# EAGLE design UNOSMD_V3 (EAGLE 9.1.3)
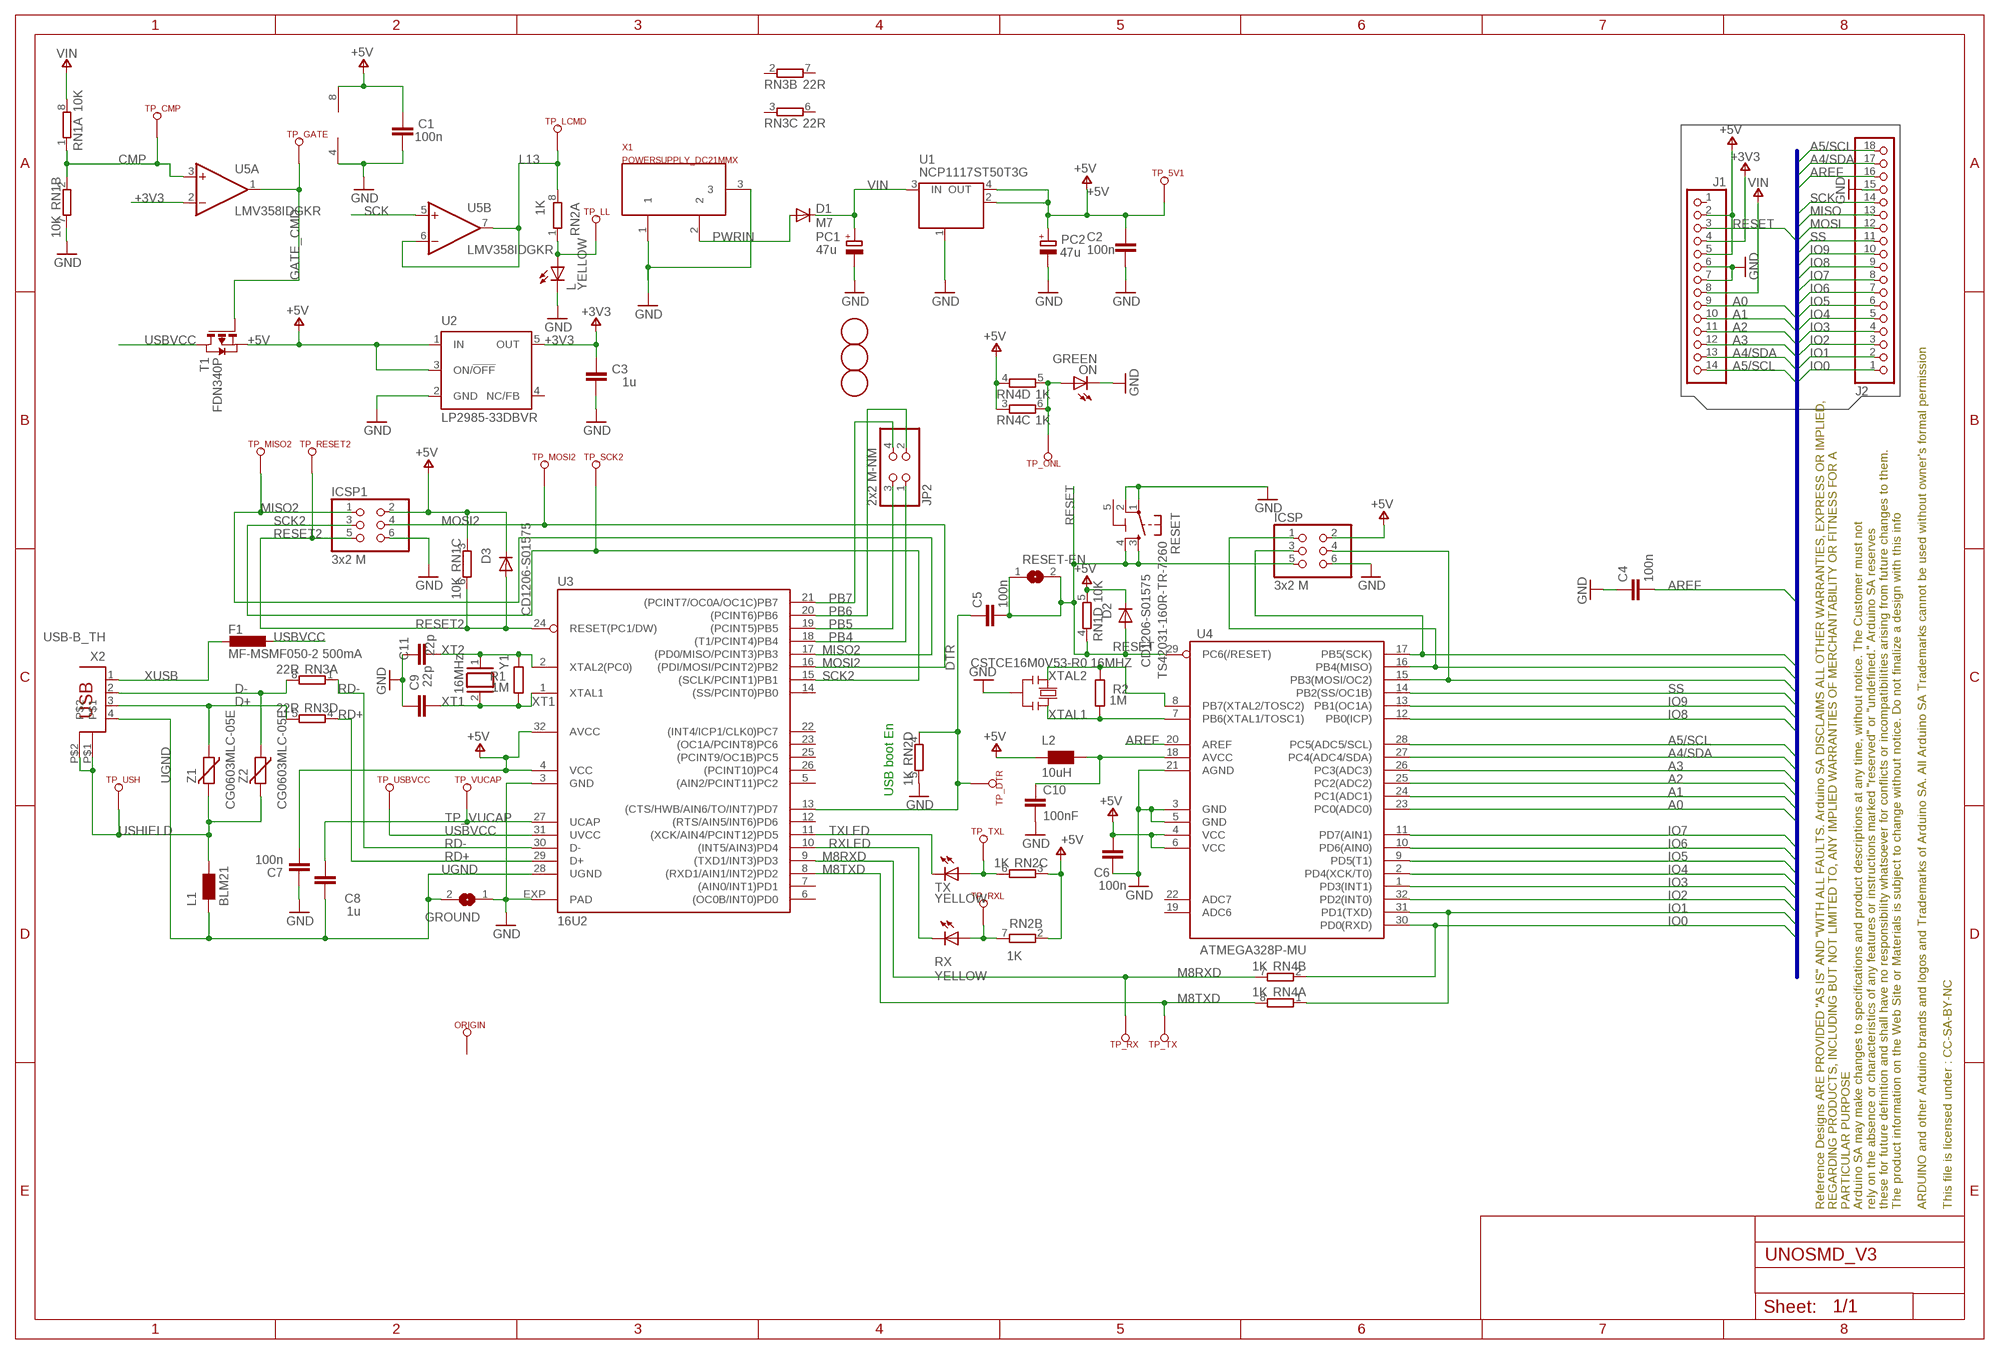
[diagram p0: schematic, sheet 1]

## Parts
C1  100n  C-EU0603-RND  [C0603-ROUND]
C2  100n  C-EU0603-RND  [C0603-ROUND]
C3  1u  C-EU0603-RND  [C0603-ROUND]
C4  100n  C-EU0603-RND  [C0603-ROUND]
C5  100n  C-EU0603-RND  [C0603-ROUND]
C6  100n  C-EU0603-RND  [C0603-ROUND]
C7  100n  C-EU0603-RND  [C0603-ROUND]
C8  1u  C-EU0603-RND  [C0603-ROUND]
C9  22p  C-EU0603-RND  [C0603-ROUND]
C10  100nF  0015_100NF_0603  [C0603-ROUND]
C11  22p  C-EU0603-RND  [C0603-ROUND]
D1  M7  DIODE-SMB  [SMB]
D2  CD1206-S01575  DIODE-MINIMELF  [MINIMELF]
D3  CD1206-S01575  DIODE-MINIMELF  [MINIMELF]
F1  MF-MSMF050-2 500mA  L-EUL1812  [L1812]
FD1  DNP  FIDUCIAL-1.5MM  [FD-1-1.5]
FD2  DNP  FIDUCIAL-1.5MM  [FD-1-1.5]
FD3  DNP  FIDUCIAL-1.5MM  [FD-1-1.5]
FRAME1  DNP  A3-FRAME-STANDARD  [FRAME]
GROUND  SJ  [SJ]
ICSP  3x2 M  PINHD-2X3  [2X03]
ICSP1  3x2 M  PINHD-2X3  [2X03]
J1  -  PINHD-1X14-CUSTOM  [1X14-CUSTOM]
J2  -  PINHD-1X18  [1X18-CUSTOM]
JP2  2x2 M-NM  PINHD-2X2  [2X02]
L  YELLOW  LEDCHIP-LED0805  [CHIP-LED0805]
L1  BLM21  WE-CBF_0805  [0805]
L2  10uH  0715_CV201210-100K  [0805]
ON  GREEN  LEDCHIP-LED0805  [CHIP-LED0805]
ORIGIN  TP_SP  [TP-SP]
PC1  47u  CPOL-EUD  [PANASONIC_D]
PC2  47u  CPOL-EUD  [PANASONIC_D]
R1  1M  R-EU_R0603  [R0603-ROUND]
R2  1M  R-EU_R0603  [R0603-ROUND]
RESET  TS42031-160R-TR-7260  TS42  [TS42]
RESET-EN  SJ  [SJ]
RN1  10K  4R-NCAY16  [CAY16]
RN2  1K  4R-NCAY16  [CAY16]
RN3  22R  4R-NCAY16  [CAY16]
RN4  1K  4R-NCAY16  [CAY16]
RX  YELLOW  LEDCHIP-LED0805  [CHIP-LED0805]
T1  FDN340P  PMOSSOT23  [SOT-23]
TP_5V1  TP_SP  [TP-SP]
TP_CMP  TP_SP  [TP-SP]
TP_DTR  TP_SP  [TP-SP]
TP_GATE  TP_SP  [TP-SP]
TP_LCMD  TP_SP  [TP-SP]
TP_LL  TP_SP  [TP-SP]
TP_MISO2  TP_SP  [TP-SP]
TP_MOSI2  TP_SP  [TP-SP]
TP_ONL  TP_SP  [TP-SP]
TP_RESET2  TP_SP  [TP-SP]
TP_RX  TP_SP  [TP-SP]
TP_RXL  TP_SP  [TP-SP]
TP_SCK2  TP_SP  [TP-SP]
TP_TX  TP_SP  [TP-SP]
TP_TXL  TP_SP  [TP-SP]
TP_USBVCC  TP_SP  [TP-SP]
TP_USH  TP_SP  [TP-SP]
TP_VUCAP  TP_SP  [TP-SP]
TX  YELLOW  LEDCHIP-LED0805  [CHIP-LED0805]
U1  NCP1117ST50T3G  MC33269ST-3.3T3  [SOT223]
U2  LP2985-33DBVR  LP2985-XXDBVR33  [SOT23-DBV]
U3  16U2  ATMEGA16U2  [ATMEL_QFN32]
U4  ATMEGA328P-MU  ATMEGAXX8-MUR  [MLF32]
U5  LMV358IDGKR  LMV358MMX  [MSOP08]
X1  POWERSUPPLY_DC21MMX  [POWERSUPPLY_DC-21MM]
X2  USB-B_TH  PN61729  [PN61729]
Y1  16MHz  XTAL/S  [QS]
Y2  CSTCE16M0V53-R0 16MHZ  RESONATORMU  [RESONATOR]
Z1  CG0603MLC-05E  VARISTORCN0603  [CT/CN0603]
Z2  CG0603MLC-05E  VARISTORCN0603  [CT/CN0603]

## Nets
+3V3: C3.2 J1.4 U2.5(OUT) U5.2(A:-IN)
+5V [usbvcc]: C1.2 C2.2 C6.2 C7.1 D2.C D3.C ICSP1.2 ICSP.2 J1.2 J1.5 L2.1 PC2.+ RN1.3 RN1.5 RN2.2 RN2.3 RN4.3 RN4.4 T1.2(S) TP_5V1.X(TESTP) U1.2(OUT) U1.4(OUT) U2.1(IN) U2.3(ON/!OFF) U3.4(VCC) U3.32(AVCC) U4.4(VCC) U4.6(VCC) U5.8(P:V+)
A0: J1.9 U4.23(PC0(ADC0))
A1: J1.10 U4.24(PC1(ADC1))
A2: J1.11 U4.25(PC2(ADC2))
A3: J1.12 U4.26(PC3(ADC3))
A4/SDA: J1.13 J2.17 U4.27(PC4(ADC4/SDA))
A5/SCL: J1.14 J2.18 U4.28(PC5(ADC5/SCL))
AREF [aref]: C4.2 J2.16 U4.20(AREF)
CMP: RN1.1 RN1.2 TP_CMP.X(TESTP) U5.3(A:+IN)
D+: RN3.5 X2.3 Z1.1
D-: RN3.8 X2.2 Z2.1
DTR: C5.1 RN2.4 TP_DTR.X(TESTP) U3.13((CTS/HWB/AIN6/TO/INT7)PD7)
GATE_CMD: T1.3(G) TP_GATE.X(TESTP) U5.1(A:OUT)
GND [gnd]: C1.1 C2.1 C3.1 C4.1 C6.1 C7.2 C9.2 C10.2 C11.2 GROUND.1 ICSP1.6 ICSP.6 J1.6 J1.7 J2.15 L.C ON.C PC1.- PC2.- RESET.1 RESET.2 RN1.7 RN2.5 U1.1(GND/ADJ) U2.2(GND) U3.3(GND) U3.EXP(PAD) U4.3(GND) U4.5(GND) U4.21(AGND) U5.4(P:V-) X1.1 X1.3 Y2.2
IO0: J2.1 RN4.2 U4.30(PD0(RXD))
IO1: J2.2 RN4.1 U4.31(PD1(TXD))
IO2: J2.3 U4.32(PD2(INT0))
IO3: J2.4 U4.1(PD3(INT1))
IO4: J2.5 U4.2(PD4(XCK/T0))
IO5: J2.6 U4.9(PD5(T1))
IO6: J2.7 U4.10(PD6(AIN0))
IO7: J2.8 U4.11(PD7(AIN1))
IO8: J2.9 U4.12(PB0(ICP))
IO9: J2.10 U4.13(PB1(OC1A))
L13: RN2.8 TP_LCMD.X(TESTP) U5.6(B:-IN) U5.7(B:OUT)
M8RXD: RN4.7 TP_RX.X(TESTP) U3.9((TXD1/INT3)PD3)
M8TXD: RN4.8 TP_TX.X(TESTP) U3.8((RXD1/AIN1/INT2)PD2)
MISO: ICSP.1 J2.13 U4.16(PB4(MISO))
MISO2: ICSP1.1 TP_MISO2.X(TESTP) U3.17((PD0/MISO/PCINT3)PB3)
MOSI: ICSP.4 J2.12 U4.15(PB3(MOSI/OC2))
MOSI2: ICSP1.4 TP_MOSI2.X(TESTP) U3.16((PDI/MOSI/PCINT2)PB2)
N$1: L.A RN2.1 TP_LL.X(TESTP)
N$3: ON.A RN4.5 RN4.6 TP_ONL.X(TESTP)
N$4 [usbvcc]: C10.1 L2.2 U4.18(AVCC)
N$35: RN2.7 RX.A TP_RXL.X(TESTP)
N$36: RN2.6 TP_TXL.X(TESTP) TX.A
PB4: JP2.1 U3.18((T1/PCINT4)PB4)
PB5: JP2.3 U3.19((PCINT5)PB5)
PB6: JP2.2 U3.20((PCINT6)PB6)
PB7: JP2.4 U3.21((PCINT7/OC0A/OC1C)PB7)
PWRIN [power]: D1.A X1.2
RD+: RN3.4 U3.29(D+)
RD-: RN3.1 U3.30(D-)
RESET: C5.2 D2.A ICSP.5 J1.3 RESET-EN.1 RESET-EN.2 RESET.3 RESET.4 RN1.4 U4.29(PC6(/RESET))
RESET2: D3.A ICSP1.5 RN1.6 TP_RESET2.X(TESTP) U3.24(RESET(PC1/DW))
RXLED: RX.C U3.10((INT5/AIN3)PD4)
SCK: ICSP.3 J2.14 U4.17(PB5(SCK)) U5.5(B:+IN)
SCK2: ICSP1.3 TP_SCK2.X(TESTP) U3.15((SCLK/PCINT1)PB1)
SS: J2.11 U4.14(PB2(SS/OC1B))
TP_VUCAP: C8.1 TP_VUCAP.X(TESTP) U3.27(UCAP)
TXLED: TX.C U3.11((XCK/AIN4/PCINT12)PD5)
UGND [gnd]: C8.2 GROUND.2 L1.1 U3.28(UGND) X2.4
USBVCC [usbvcc]: F1.1 T1.1(D) TP_USBVCC.X(TESTP) U3.31(UVCC)
USHIELD [gnd]: L1.2 TP_USH.X(TESTP) X2.P$1 X2.P$2 Z1.2 Z2.2
VIN [power]: D1.C J1.8 PC1.+ RN1.8 U1.3(IN)
XT1: C9.1 R1.1 U3.1(XTAL1) Y1.2
XT2: C11.1 R1.2 U3.2(XTAL2(PC0)) Y1.1
XTAL1: R2.1 U4.7(PB6(XTAL1/TOSC1)) Y2.3
XTAL2: R2.2 U4.8(PB7(XTAL2/TOSC2)) Y2.1
XUSB [usbvcc]: F1.2 X2.1
Unconnected: J1.1 ORIGIN.X(TESTP) RN3.2 RN3.3 RN3.6 RN3.7 U2.4(NC/FB) U3.5((AIN2/PCINT11)PC2) U3.6((OC0B/INT0)PD0) U3.7((AIN0/INT1)PD1) U3.12((RTS/AIN5/INT6)PD6) U3.14((SS/PCINT0)PB0) U3.22((INT4/ICP1/CLK0)PC7) U3.23((OC1A/PCINT8)PC6) U3.25((PCINT9/OC1B)PC5) U3.26((PCINT10)PC4) U4.19(ADC6) U4.22(ADC7)

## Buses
B$1

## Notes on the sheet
- USB boot En

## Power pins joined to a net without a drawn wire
5-GND: RESET.5(5-GND)

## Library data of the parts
C1-C9 C11 = SmartPrj:C-EU: CAPACITOR, European symbol
C10 = Condensatori:0015_100NF_0603: 100nF 0603; CASE: 0603; MONTHLY_USAGE: _____; PART_NUMBER: 100nF_0603; PRICE: _____; SUPPLIER: _____; TYPE: Condensatori
D1-D3 = diode:DIODE-: DIODE
F1 = rcl:L-EU: INDUCTOR, European symbol
FD1-FD3 = Arduino-utility:FIDUCIAL: Fiducial mount; DATASHEET: DNP; DISTRIBUTOR-LINK: DNP; DISTRIBUTOR-PN: DNP; MANUFACTURER: DNP; MANUFACTURER-PN: DNP
FRAME1 = Arduino-utility:A3-FRAME: Schematic frame; CODE-ARDUINO: DNP; DATASHEET: DNP; DISTRIBUTOR-LINK: DNP; DISTRIBUTOR-PN: DNP; MANUFACTURER: DNP; MANUFACTURER-PN: DNP
GROUND RESET-EN = jumper:SJ: SMD solder JUMPER
ICSP ICSP1 = SmartPrj:PINHD-2X3: PIN HEADER
J1 = Arduino-connectors:PINHD-1X14: PIN HEADER; DATASHEET: -; DISTRIBUTOR-PN: -; MANUFACTURER: -; MANUFACTURER-PN: -
J2 = Arduino-connectors:PINHD-1X18; DATASHEET: -; DISTRIBUTOR-LINK: -; DISTRIBUTOR-PN: -; MANUFACTURER-PN: -; MANUFCATURER: -
JP2 = SmartPrj:PINHD-2X2: PIN HEADER
L ON RX TX = led:LED: LED
L1 = wuerth-elektronik:WE-CBF: SMD EMI Suppression Ferrite Beads
L2 = Induttanze:0715_CV201210-100K: 10uH 0805; CASE: 0805; MONTHLY_USAGE: _____; PART_NUMBER: CV201210-100K; PRICE: _____; SUPPLIER: _____; TYPE: Induttanze
ORIGIN TP_5V1 TP_CMP TP_DTR TP_GATE TP_LCMD TP_LL TP_MISO2 TP_MOSI2 TP_ONL TP_RESET2 TP_RX TP_RXL TP_SCK2 TP_TX TP_TXL TP_USBVCC TP_USH TP_VUCAP = SmartPrj:TP_SP
PC1 PC2 = rcl:CPOL-EU: POLARIZED CAPACITOR, European symbol
R1 R2 = SmartPrj:R-EU_: RESISTOR, European symbol
RESET = SmartPrj:TS42: TS42 Dongnan Electronics Tact switch VDC 12V - 50mA
RN1-RN4 = resistor-dil:4R-N: Array Chip Resistor Source: RS Component / Phycomp
T1 = zetex:PMOSSOT23: MOS FET
U1 = linear:MC33269ST*: Adjustable Output Low Dropout Voltage Regulator 800 mA Source: http://www.onsemi.com/pub/Collateral/MC33269-D.PDF
U2 = SmartPrj:LP2985-XXDBVR: ULTRALOW-POWER 50-mA LOW-DROPOUT LINEAR REGULATORS 50-mA Low-Dropout Regulator Source: http://focus.ti.com/lit/ds/symlink/tps77001.pdf
U3 = Arduino-ucs&SoCs:ATMEGA16U2: AVR AVR® ATmega Microcontroller IC 8-Bit 16MHz 16KB (8K x 16) FLASH 32-VQFN (5x5); DATASHEET: http://www.digikey.com/product-detail/en/atmel/ATMEGA16U2-MU/ATMEGA16U2-MU-ND/2050821; DISTRIBUTOR-LINK: http://www.digikey.com/product-detail/en/atmel/ATMEGA16U2-MU/ATMEGA16U2-MU-ND/2050821; DISTRIBUTOR-PN: ATMEGA16U2-MU-ND; MANUFACTURER: ATMEL; MANUFACTURER-PN: ATMEGA16U2-MU
U4 = SmartPrj:ATMEGAXX8: MICROCONTROLLER 8 Kbytes FLASH 1 kbytes SRAM 512 bytes EEPROM USART 6-channel 10 bit ADC 2-channel 8 bit ADC Source: avr.lbr
U5 = linear:LMV358?*: Dual General Purpose, Low Voltage, Rail-to-Rail Output Operational Amplifiers Source: http://www.national.com/mpf/LM/LMV321.html http://www.national.com/dt/lmv_qual.pdf
X1 = SmartPrj:POWERSUPPLY_DC21MM
X2 = SmartPrj:PN61729: BERG USB connector
Y1 = SmartPrj:XTAL/S: CRYSTAL
Y2 = SmartPrj:RESONATOR
Z1 Z2 = varistor:VARISTOR: VARISTOR

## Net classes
0 default: width 0.254 mm, clearance 0.254 mm
1 power: width 0.61 mm, drill 0.61 mm, clearance 0.254 mm
2 gnd: width 0.305 mm, drill 0.559 mm, clearance 0.254 mm
3 usbvcc: width 0.508 mm, drill 0.61 mm, clearance 0.254 mm
4 aref: width 0.406 mm, drill 0.61 mm, clearance 0.254 mm

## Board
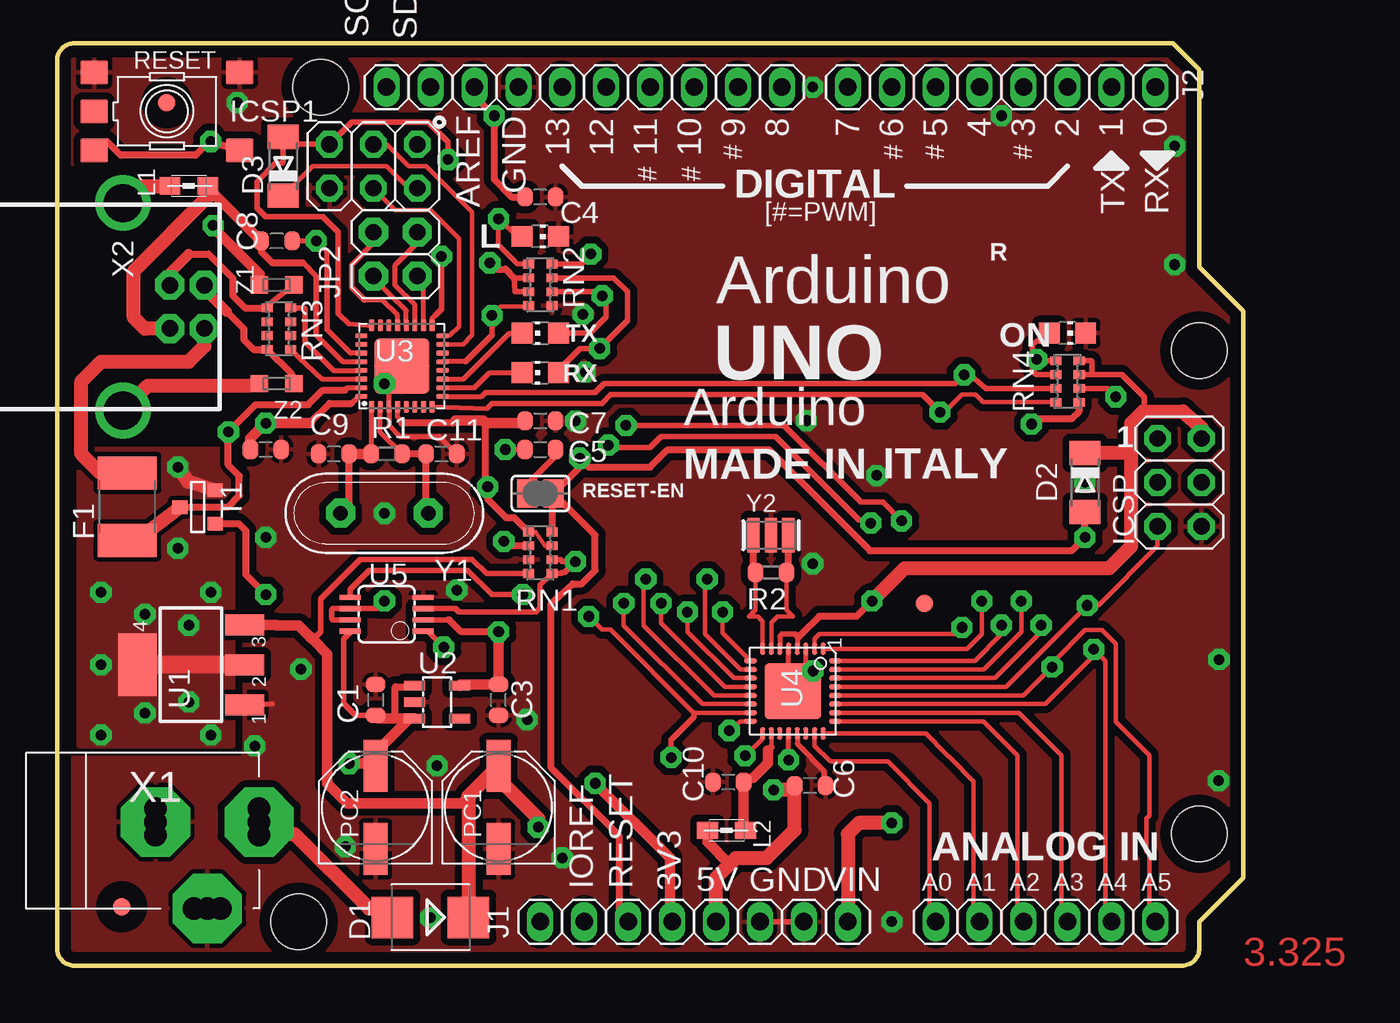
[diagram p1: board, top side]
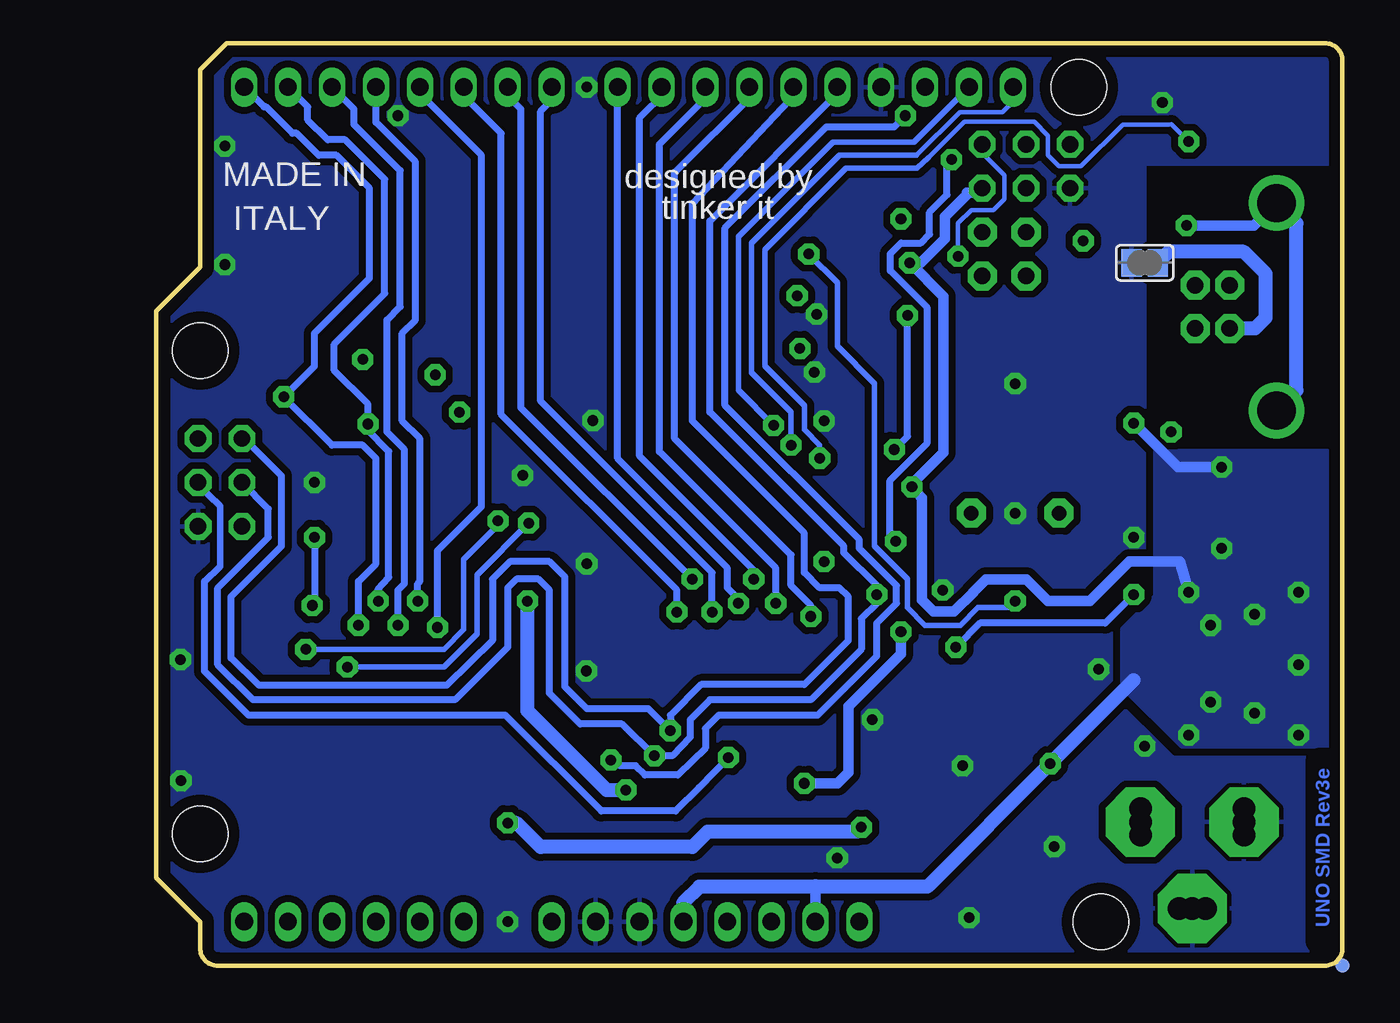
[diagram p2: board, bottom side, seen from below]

Size 68.58 x 53.34 mm. Coordinates in mm from the lower left corner, seen from the top.
Outline: 0,1 arc90 1,0 65.04,0 arc90 66.04,1 66.04,2.54 68.58,5.08 68.58,37.85 66.04,40.39 66.04,51.82 64.52,53.34 1,53.34 arc90 0,52.34
Outline: 0,52.32 0,1.02
Copper layers (1*16): Top 0.035mm / dielectric 1.5mm / Bottom 0.035mm
Design rules "ArduinoUno *": minimum track width 10mil, minimum drill 22mil, track to track 10mil, track to pad 10mil, pad to pad 10mil, via to via 12mil, smd to smd 8mil, copper to edge 26mil, drill to drill 12mil, minimum pad ring 10mil, minimum via ring 12mil, stop-mask expansion 1mil, vias tented up to drill 30mil, thermal gap 10mil
Holes 3.2 mm at 66.04,35.56 66.04,7.62 15.24,50.8 13.97,2.54
bKeepout: area -0.1,3.2 to 1.9,11
bRestrict: 5 lines
vRestrict: area 22.9,44.1 to 24.6,49.1; area 25.4,45.5 to 27.1,49.1; area 28.4,45.3 to 29.6,48.8; area 31,45.3 to 32.1,48.8; area 33.5,45.3 to 34.7,48.8; area 36.1,45.3 to 37.2,48.8; area 38.7,47.2 to 39.9,48.8; area 40.3,45.1 to 47.6,46.9; area 60.3,44.2 to 61.7,46.7; area 62.9,44.2 to 64.3,46.7; area 61.3,35.8 to 64.8,37.2; area 0.6,21.8 to 2,30.1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

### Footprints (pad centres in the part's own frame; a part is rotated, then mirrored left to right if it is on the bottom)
C0603-ROUND = smd 0.898 x 1.1: 1 -0.889,0; 2 0.889,0
SMB = smd 2.4 x 2.4: A 2.2,0; C -2.2,0
MINIMELF = smd 1.4 x 1.8: A 1.7,0; C -1.7,0
L1812 = smd 1.9 x 3.4: 1 -1.95,0; 2 1.95,0
FD-1-1.5 = smd 1.016 x 1.016: P$1 0,0
SJ = smd 1.168 x 1.6: 1 -0.762,0; 2 0.762,0
2X03 = drill 0.95 pad 1.55 octagon: 1 -2.54,-1.27; 2 -2.54,1.27; 3 0,-1.27; 4 0,1.27; 5 2.54,-1.27; 6 2.54,1.27
1X14-CUSTOM = drill 1.016 pad 1.27 long: 1 -17.78,0; 2 -15.24,0; 3 -12.7,0; 4 -10.16,0; 5 -7.62,0; 6 -5.08,0; 7 -2.54,0; 8 0,0; 9 5.08,0; 10 7.62,0; 11 10.16,0; 12 12.7,0; 13 15.24,0; 14 17.78,0
1X18-CUSTOM = drill 1.016 pad 1.27 long: 1 -17.78,0; 2 -15.24,0; 3 -12.7,0; 4 -10.16,0; 5 -7.62,0; 6 -5.08,0; 7 -2.54,0; 8 0,0; 9 3.81,0; 10 6.35,0; 11 8.89,0; 12 11.43,0; 13 13.97,0; 14 16.51,0; 15 19.05,0; 16 21.59,0; 17 24.13,0; 18 26.67,0
2X02 = drill 0.95 pad 1.676 octagon: 1 -1.27,-1.27; 2 -1.27,1.27; 3 1.27,-1.27; 4 1.27,1.27
CHIP-LED0805 = smd 1.2 x 1.2: A 0,-1.05; C 0,1.05
0805 = smd 1.2 x 1: 1 -1.1,0; 2 1.1,0
TP-SP = smd 0.8 x 0.8 bottom: X 0,0
PANASONIC_D = smd 3 x 1.4: + 2.4,0; - -2.4,0
R0603-ROUND = smd 0.898 x 1.1: 1 -0.889,0; 2 0.889,0
TS42 = smd 1.6 x 1.4: 1 -4.2,2.25; 2 4.2,2.25; 3 -4.2,-2.25; 4 4.2,-2.25; 5 -4.2,0
CAY16 = smd 0.5 x 0.65: 1 -1.2,-0.675; 2 -0.4,-0.675; 3 0.4,-0.675; 4 1.2,-0.675; 5 1.2,0.675; 6 0.4,0.675; 7 -0.4,0.675; 8 -1.2,0.675
SOT-23 = smd 0.787 x 0.889: 1 0.025,-1.016; 2 -0.94,1.016; 3 0.991,1.016
SOT223 = smd 1.219 x 2.235: 1 -2.311,-3.099; 2 0,-3.099; 3 2.311,-3.099 | smd 3.6 x 2.2: 4 0,3.099
SOT23-DBV = smd 0.55 x 1.2: 1 -0.95,-1.3; 2 0,-1.3; 3 0.95,-1.3; 4 0.95,1.3; 5 -0.95,1.3
ATMEL_QFN32 = smd 0.711 x 0.305: 1 -2.351,1.75; 2 -2.351,1.25; 3 -2.351,0.75; 4 -2.351,0.25; 5 -2.351,-0.25; 6 -2.351,-0.75; 7 -2.351,-1.25; 8 -2.351,-1.75; 17 2.351,-1.75; 18 2.351,-1.25; 19 2.351,-0.75; 20 2.351,-0.25; 21 2.351,0.25; 22 2.351,0.75; 23 2.351,1.25; 24 2.351,1.75 | smd 0.305 x 0.711: 9 -1.75,-2.351; 10 -1.25,-2.351; 11 -0.75,-2.351; 12 -0.25,-2.351; 13 0.25,-2.351; 14 0.75,-2.351; 15 1.25,-2.351; 16 1.75,-2.351; 25 1.75,2.351; 26 1.25,2.351; 27 0.75,2.351; 28 0.25,2.351; 29 -0.25,2.351; 30 -0.75,2.351; 31 -1.25,2.351; 32 -1.75,2.351 | smd 3.2 x 3.2: EXP 0,0
MLF32 = smd 0.7 x 0.28: 1 -2.45,1.75; 2 -2.45,1.25; 3 -2.45,0.75; 4 -2.45,0.25; 5 -2.45,-0.25; 6 -2.45,-0.75; 7 -2.45,-1.25; 8 -2.45,-1.75; 17 2.45,-1.75; 18 2.45,-1.25; 19 2.45,-0.75; 20 2.45,-0.25; 21 2.45,0.25; 22 2.45,0.75; 23 2.45,1.25; 24 2.45,1.75 | smd 0.28 x 0.7: 9 -1.75,-2.45; 10 -1.25,-2.45; 11 -0.75,-2.45; 12 -0.25,-2.45; 13 0.25,-2.45; 14 0.75,-2.45; 15 1.25,-2.45; 16 1.75,-2.45; 25 1.75,2.45; 26 1.25,2.45; 27 0.75,2.45; 28 0.25,2.45; 29 -0.25,2.45; 30 -0.75,2.45; 31 -1.25,2.45; 32 -1.75,2.45 | smd 3.254 x 3.254: 33 0,0
MSOP08 = smd 0.3 x 1.2: 1 -0.976,-2.113; 2 -0.326,-2.113; 3 0.324,-2.113; 4 0.974,-2.113; 5 0.974,2.112; 6 0.324,2.112; 7 -0.326,2.112; 8 -0.976,2.112
POWERSUPPLY_DC-21MM = drill 1.3 pad 4 octagon: 1 -5.08,-3.353; 2 -0.076,-6.35; 3 -0.076,-0.356 | drill 1.3: 4 -5.08,-4.115; 5 -5.08,-2.591; 6 -0.838,-0.356; 7 0.686,-0.356; 8 -0.838,-6.35; 9 0.686,-6.35
PN61729 = drill 0.95 pad 1.676 octagon: 1 1.25,4.71; 2 -1.25,4.71; 3 -1.25,2.71; 4 1.25,2.71 | drill 2.2: P$1 -6,0; P$2 6,0
QS = drill 0.85 pad 1.676 octagon: 1 -2.54,0; 2 2.54,0
RESONATOR = smd 0.7 x 2: 1 -1,0; 2 0,0; 3 1,0
CT/CN0603 = smd 1 x 1: 1 -1,0; 2 1,0

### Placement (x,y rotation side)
C1  18.41,15.37 270 top
C2  12.06,29.84 180 top
C3  25.53,15.37 90 top
C4  27.94,44.45 180 top
C5  27.94,29.84 0 top
C6  43.54,10.41 180 top
C7  27.94,31.5 0 top
C8  12.7,41.91 180 top
C9  16,29.59 180 top
C10  38.81,10.62 180 top
C11  22.23,29.59 0 top
D1  21.59,2.79 180 top
D2  59.44,27.94 270 top
D3  13.08,46.23 90 top
F1  4.06,26.54 90 top
FD1  6.35,49.91 0 top
FD2  50.16,20.93 0 top
FD3  3.73,3.41 0 top
FRAME1  not placed on the board
GROUND  11.43,40.64 0 bottom
ICSP  64.9,27.94 270 top
ICSP1  18.29,46.23 180 top
J1  45.72,2.54 0 top
J2  45.72,50.8 180 top
JP2  19.56,41.15 90 top
L  27.94,42.16 270 top
L1  7.62,45.09 180 top
L2  38.71,7.82 0 top
ON  58.42,36.58 270 top
ORIGIN  0,0 0 top
PC1  25.53,9.14 90 top
PC2  18.41,9.14 90 top
R1  19.05,29.59 0 top
R2  41.27,22.73 180 top
RESET  6.35,49.4 0 top
RESET-EN  27.94,27.3 0 top
RN1  27.94,23.88 90 top
RN2  27.94,39.37 270 top
RN3  12.83,36.83 90 top
RN4  58.42,33.78 90 top
RX  27.94,34.29 90 top
T1  8.13,26.54 270 top
TP_5V1  66.17,30.48 0 top
TP_CMP  29.97,23.37 0 top
TP_DTR  25.91,29.84 0 top
TP_GATE  12.06,21.46 0 top
TP_LCMD  18.92,21.08 0 top
TP_LL  25.53,43.18 0 top
TP_MISO2  20.83,47.5 0 top
TP_MOSI2  18.29,44.96 0 top
TP_ONL  56.64,35.05 0 top
TP_RESET2  15.75,47.5 0 top
TP_RX  52.45,34.16 0 top
TP_RXL  31.37,35.69 0 top
TP_SCK2  18.29,47.5 0 top
TP_TX  51.05,32 0 top
TP_TXL  31.37,38.73 0 top
TP_USBVCC  9.91,30.86 0 top
TP_USH  9.02,42.8 0 top
TP_VUCAP  14.99,41.91 0 top
TX  27.94,36.58 90 top
U1  7.75,17.4 90 top
U2  21.97,15.24 270 top
U3  19.94,34.67 90 top
U4  42.55,15.88 270 top
U5  19.05,20.32 90 top
X1  5.33,8.38 90 top
X2  3.81,38.1 270 top
Y1  18.92,26.16 180 top
Y2  41.27,24.89 0 top
Z1  12.7,39.37 180 top
Z2  12.7,33.66 180 top

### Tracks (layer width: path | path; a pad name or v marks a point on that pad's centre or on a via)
+3V3  (via drill 0.61)
  Top 0.305: 22.61,19.99 U5.2
  Top 0.406: 22.61,19.99 22.68,19.99 23.37,19.3 v25.53,19.3
  Top 0.61: v31.11,10.54 35.43,6.22 35.43,2.67 J1.4 | U2.5 23.34,16.26 C3.2 v25.53,19.3
  Bottom 0.61: v31.11,10.54 29.21,10.54 28.57,11.18 28.57,14.99 25.53,18.03 v25.53,19.3
+5V  (via drill 0.61)
  Top 0.254: 27.32,25.02 RN1.5 27.65,25.08 28.23,24.28 RN1.3 | ICSP1.2 20.32,44.96 19.05,46.23 14.78,46.23 D3.C
  Top 0.279: U3.4 19.69,31.75 19.94,31.37 | U3.32 17.43,32.92 17.02,32.51 | 41.91,19.18 41.8,19.06 U4.6 | 42.8,19.05 U4.4
  Top 0.305: 59.82,34.18 61.58,34.18 62.87,32.89 62.87,32.05 | 59.82,34.18 RN4.3 | RN4.4 59.76,34.98 59.82,34.92 59.82,34.18 | RN2.2 26.43,39.77 26.47,38.97 RN2.3 | U5.8 16.98,19.3 16.57,18.9 16.57,15.18 17.27,14.48 C1.2 | 42.8,19.05 42.67,19.18 41.91,19.18
  Top 0.406: 26.43,39.77 25.93,40.28 25.53,40.26 v25.02,40.64 | RN1.5 26.43,25.91 25.96,25.91 24.89,26.97 v24.89,27.69 24.77,28.19 24.77,31.38 | 19.94,31.37 22.89,31.37 23.03,31.51 | 17.02,32.51 15.75,32.51 14.61,31.37 | U2.1 20.61,16.13 19.56,16.13 19.56,14.29 | 42.8,19.05 42.93,19.05 44.07,20.19 46.23,20.19 v47.12,21.08
  Top 0.508: 11.02,17.42 U1.2 | TP_5V1.X 66.04,30.48
  Top 0.61: 23.03,31.51 24.64,31.51 24.77,31.38 26.94,31.38 C7.1 | 11.05,29.72 C2.2 11.18,30.48 v12.06,31.37 14.61,31.37 | v16.89,11.68 18.78,11.68 PC2.+ 18.41,12.32 20.39,14.29 U2.3 19.56,14.29 18.6,14.29 C1.2 | L2.1 37.61,7.14 38.89,5.87
  Top 0.813: 66.17,30.44 TP_5V1.X 66.17,31.11 65.1,32.05 62.87,32.05 62.79,32.05 62.1,31.37 62.1,29.46 | 62.1,29.46 62.1,24.26 60.83,22.99 49.02,22.99 v47.12,21.08 | T1.2 7.57,27.99 v6.99,28.83 | D2.C 61.93,29.64 62.1,29.46 | J1.5 38.1,5.08 38.89,5.87 39.24,6.22 41.02,6.22 42.65,7.85 C6.2 42.39,10.16 v41.43,10.16
  Top 1.016: U1.4 5.84,17.4 5.87,17.42 11.02,17.42
  Bottom 0.61: ICSP1.2 21.08,44.7 21.72,44.7 21.72,44.58 22.99,43.31 22.99,42.04 24.38,40.64 v25.02,40.64 23.07,38.69 23.07,29.68 24.89,27.85 v24.89,27.69 24.31,27.05 24.31,21.13 23.65,20.47 22.45,20.47 21.34,21.59 21.36,21.59 20.62,22.33 18.26,22.33 17.02,21.08 14.61,21.08 12.32,23.37 9.4,23.37 v8.89,21.59 | J1.2 30.48,4.7 30.61,4.57 | v12.06,31.37 9.53,28.83 v6.99,28.83
  Bottom 0.813: J1.5 38.12,3.63 37.19,4.57 30.61,4.57 24,4.57 v16.89,11.68 12.06,16.51 | v47.12,21.08 47.12,14.73 42.55,10.16 v41.43,10.16
  other vias: 2.54,21.59 5.08,20.32 6.99,24.13 2.54,13.34 5.08,14.61 2.54,17.4 8.89,13.34 7.62,15.24 7.62,19.68
  pour Bottom (isolate 0.406, no thermals): 0.89,29.72 10.79,29.72 10.79,21.34 12.7,19.43 12.7,16.13 9.27,12.7 0.89,12.7
  pour Top (no thermals): 1.27,12.7 1.27,29.84 10.16,29.84 10.16,12.7
A0
  Top 0.254: J1.9 50.44,3 50.44,9.4 48.03,11.81 44.7,11.81 43.8,12.72 U4.23
A1
  Top 0.254: J1.10 52.98,3 52.98,10.67 51.7,11.95 51.44,12.22 50.23,13.43 U4.24
A2
  Top 0.254: J1.11 55.52,3 55.52,12.17 53.57,14.12 U4.25
A3
  Top 0.254: J1.12 58.06,3 58.06,12.17 55.61,14.62 U4.26
A4/SDA  (via drill 0.61)
  Top 0.254: J1.13 60.6,3 60.6,17.63 v59.94,18.29 59.94,17.93 57.14,15.12 U4.27
  Top 0.305: v32.89,31.24 42.04,31.24 46.48,26.8 47.75,26.8 v48.83,25.72 49.02,25.65
  Bottom 0.305: v48.83,25.72 48.9,25.65 48.9,25.4 50.8,23.5 50.8,19.43 51.94,18.29 v59.94,18.29 | v32.89,31.24 34.92,33.27 34.92,42.16 29.46,47.62 24.77,47.62 J2.17
A5/SCL  (via drill 0.61)
  Top 0.254: J1.14 63.14,3 63.14,6.45 62.99,6.6 62.99,8.51 63.14,8.66 63.14,12.17 61.21,14.1 61.21,18.59 60.4,19.41 59.44,19.41 57.71,17.68 57.71,17.45 v57.53,17.27 55.88,15.62 U4.28
  Top 0.305: v31.88,30.1 31.88,29.97 34.29,29.97 34.92,30.61 41.53,30.61 46.35,25.78 46.86,25.78 v47.05,25.59
  Bottom 0.254: 24.64,46.86 22.12,49.35 19.65,49.35 19,50 19,50.75 J2.18
  Bottom 0.305: v31.88,30.1 31.88,32 34.16,34.29 34.16,41.78 29.08,46.86 24.64,46.86 | v47.05,25.59 50.04,22.61 50.04,19.18 51.94,17.27 v57.53,17.27
AREF  (via drill 0.61)
  Top 0.254: 23.88,50.55 J2.16
  Top 0.279: 42.3,12.07 U4.20
  Top 0.305: v42.29,11.89 42.3,12.07
  Top 0.406: 23.88,50.55 v25.27,49.15 25.27,45.47 26.29,44.45 C4.2
  Bottom 0.406: v25.27,49.15 25.91,48.51 29.84,48.51 35.69,42.67 35.69,32.38 27.94,24.64 27.94,24.13 25.78,21.97 25.78,20.95 26.92,19.81 26.92,17.91 30.35,14.48 36.07,14.48 36.83,13.72 36.83,12.57 38.43,11.02 40.34,11.02 40.87,11.56 41.78,11.56 v42.29,11.89
CMP  (via drill 0.61)
  Top 0.305: U5.3 23.04,20.64 23.24,20.45 27.69,20.45 27.94,20.7 27.94,22 RN1.1 29.15,22.68 29.21,22.73 29.34,22.73 TP_CMP.X 29.21,23.37 29.1,23.48 RN1.2
  other vias: 29.97,23.37
D+
  Top 0.305: Z1.1 12.1,38.1 RN3.5
  Top 0.406: 7.62,41.15 8.76,41.15 10.16,39.75 10.16,38.73 10.87,38.03 RN3.5
  Top 0.61: X2.3 6.52,40.05 7.62,41.15
  Bottom 0.61: 6.5,39.37 X2.3
D-
  Top 0.406: 9.82,37.81 10.79,36.83 10.79,36.2 11.36,35.63 RN3.8 13.49,34.29 Z2.1
  Top 0.61: X2.2 8.53,39.1 9.82,37.81
  Bottom 0.305: X2.2
DTR  (via drill 0.61)
  Top 0.254: v25.15,37.59 25.65,38.1 27.2,38.1
  Top 0.279: 23.62,34.92 U3.13
  Top 0.305: TP_DTR.X C5.1 | 27.2,38.1 RN2.4 | 23.62,34.92 25.15,36.45 v25.15,37.59
  Bottom 0.406: TP_DTR.X 25.15,30.61 v25.15,37.59
  other vias: 25.91,29.84
GATE_CMD  (via drill 0.61)
  Top 0.305: U5.1 21.42,19.34 v22.35,18.41
  Top 0.406: T1.3 10.52,25.55 10.92,25.15 10.92,22.61 TP_GATE.X
  Bottom 0.406: v22.35,18.41 20.95,19.81 13.72,19.81 TP_GATE.X
  other vias: 12.06,21.46
GND  (via drill 0.61)
  Top 0.279: C11.2 22.1,30.61 19.81,30.61 19.19,31.23 U3.3 19.19,33.39 v18.92,33.66 | 43.3,17.46 U4.3 | 42.3,17.27 U4.5 | U4.21 42.8,12.83 44.32,11.3
  Top 0.305: J1.6 J1.7 | U1.1 12.45,15.14 | 19.19,33.52 v18.92,33.66 U3.EXP | 43.3,17.46 v43.71,17.04 43.69,17.02 42.55,17.02 42.3,17.27 | 44.32,11.3 C6.1
  Bottom 0.305: GROUND.1 10.79,40.64
  other vias: 29.21,6.22 27.18,14.22 16.66,6.88 30.53,34.32 54.61,49.15 30.4,37.67 11.43,12.7 43.69,23.24 29.97,31.5 43.69,50.8 48.26,2.54 59.44,27.94 21.59,2.77 67.16,10.69 64.62,47.4 12.06,24.77 67.18,17.7 23.11,21.72 10.41,49.91 47.4,28.35 18.92,26.16 43.33,31.52 21.97,11.56 14.1,17.14 64.62,40.54
  pour Bottom (isolate 0.406, rank 2): 0.64,52.7 67.69,52.7 67.94,52.45 67.94,0.64 0.89,0.64 0.64,0.89 0.64,30.1 11.43,30.1 11.43,46.35 0.64,46.35
  pour Top (isolate 0.406, rank 2): 0.64,52.7 67.94,52.7 67.94,0.64 0.64,0.64 0.51,30.48 11.43,30.48 11.43,46.35 0.64,46.35
IO0  (via drill 0.61)
  Top 0.254: U4.30 54.22,16.62 56.9,19.3 v56.9,19.68
  Top 0.305: RN4.2 60.73,33.38 v61.21,32.89
  Bottom 0.406: J2.1 62.36,49.66 62.23,49.66 60.71,48.13 60.45,48.13 59.18,46.86 58.17,46.86 56.26,44.96 56.26,39.75 59.44,36.58 59.44,34.67 v61.21,32.89 58.42,30.1 56.64,30.1 55.88,29.34 55.88,23.24 56.9,22.23 v56.9,19.68
IO1  (via drill 0.61)
  Top 0.254: U4.31 53.57,17.12 55.75,19.3 v55.75,21.08
  Top 0.406: RN4.1 59.09,32.04 58.67,31.62 56.64,31.62 v56.34,31.32
  Bottom 0.406: J2.2 59.82,49.66 59.82,48.9 58.67,47.75 57.66,47.75 55.37,45.47 55.37,38.86 58.29,35.94 58.29,34.42 56.34,32.46 v56.34,31.32 56.39,31.11 56.39,30.99 55.14,29.74 55.14,22.45 55.75,21.79 v55.75,21.08
IO2  (via drill 0.61)
  Top 0.254: U4.32 53.06,17.62 54.61,19.18 v54.61,19.68
  Bottom 0.406: J2.3 57.15,49.53 57.15,48.64 54.48,45.97 54.48,38.1 55.24,37.34 55.24,30.86 54.23,29.84 54.23,22.1 54.61,21.72 v54.61,19.68
IO3  (via drill 0.61)
  Top 0.254: U4.1 52.62,18.32 53.47,19.18 v53.47,21.08
  Bottom 0.406: J2.4 55.88,48.77 53.59,46.48 53.59,37.34 54.36,36.58 54.36,31.5 53.34,30.48 53.34,22.23 53.47,22.1 v53.47,21.08
IO4  (via drill 0.61)
  Top 0.254: U4.2 43.8,18.9 44.07,19.18 51.94,19.18 v52.32,19.56
  Bottom 0.406: J2.5 53.21,50.29 49.78,46.86 49.78,26.54 52.32,24 v52.32,19.56
IO5  (via drill 0.61)
  Top 0.254: U4.9 38.48,19.24 v38.48,20.45
  Bottom 0.406: J2.6 50.8,50.29 48.64,48.13 48.64,31.88 38.48,21.72 v38.48,20.45
IO6  (via drill 0.61)
  Top 0.254: U4.10 39.52,17.12 37.47,19.18 37.47,22.23 v37.59,22.35
  Bottom 0.406: J2.7 48.26,50.29 47.5,49.53 47.5,32.26 v37.59,22.35
IO7  (via drill 0.61)
  Top 0.254: U4.11 39.13,16.62 36.45,19.3 v36.45,20.45
  Bottom 0.406: J2.8 45.72,50.04 46.35,49.4 46.35,32.64 36.45,22.73 v36.45,20.45
IO8  (via drill 0.61)
  Top 0.254: U4.12 38.61,16.12 34.92,19.81 v34.92,20.95
  Bottom 0.254: 41.91,50.55 J2.9
  Bottom 0.406: 41.91,50.55 41.91,29.34 35.56,22.99 35.56,21.84 34.92,21.21 v34.92,20.95
IO9  (via drill 0.61)
  Top 0.254: U4.13 37.97,15.62 33.91,19.68 33.91,22.1 34.04,22.23 v34.04,22.35
  Bottom 0.254: 39.12,50.55 J2.10
  Bottom 0.406: 39.12,50.55 40.64,49.02 40.64,29.46 34.04,22.86 v34.04,22.35
L13  (via drill 0.61)
  Top 0.305: U5.7 15.95,19.99 15.88,20.07 15.88,20.57 15.95,20.64 U5.6 18.48,20.64 TP_LCMD.X | RN2.8 30.28,40.57 v30.86,41.15
  Bottom 0.305: v30.86,41.15 29.21,39.5 29.21,35.81 27.05,33.66 27.05,24.26 25.15,22.35 25.15,20.7 24.13,19.68 22.1,19.68 21.08,20.7 19.3,20.7 TP_LCMD.X
  other vias: 18.92,21.08
M8RXD  (via drill 0.61)
  Top 0.279: U3.9 24.54,32.92 24.77,33.15
  Top 0.305: RN4.7 53.7,33.38 52.79,34.16 TP_RX.X 51.94,33.66 31.62,33.66 31.11,33.15 24.77,33.15
  other vias: 52.45,34.16
M8TXD  (via drill 0.61)
  Top 0.254: RN4.8 53.52,32.58 53.09,33.02 52.32,33.02 51.31,32 TP_TX.X
  Top 0.279: U3.8 24.86,32.22 25.15,32.51
  Top 0.305: 25.15,32.51 31.5,32.51 32,33.02 50.04,33.02 TP_TX.X
  other vias: 51.05,32
MISO  (via drill 0.61)
  Top 0.254: U4.16 39.52,14.12 v38.86,13.59
  Bottom 0.254: 31.5,50.55 J2.13
  Bottom 0.406: 31.5,50.55 37.59,44.07 37.59,31.5 31.11,25.02 31.11,22.73 30.23,21.84 29.08,21.84 28.57,21.34 28.57,18.8 31.11,16.26 37.08,16.26 38.86,14.48 v38.86,13.59 40.13,14.86 43.69,14.86 44.96,16.13 44.96,22.48 45.85,23.37 48.13,23.37 49.15,22.35 49.15,18.8 51.79,16.2 62.64,16.2 64.26,17.78 64.26,21.34 61.34,24.26 61.34,28.32 63.45,30.43 ICSP.1
MISO2  (via drill 0.61)
  Top 0.254: v22.23,41.02 22.23,39.5
  Top 0.279: 21.84,37.59 21.69,37.44 U3.17
  Top 0.305: v22.23,41.02 22.23,37.97 21.84,37.59
  Bottom 0.254: v22.23,41.02 22.23,42.93 21.46,43.69 20.19,43.69 19.56,44.32 19.56,45.72 20.83,46.99 TP_MISO2.X
MOSI  (via drill 0.61)
  Top 0.254: 36.81,14.62 U4.15 | 36.81,14.62 32,19.43 31.5,19.43 v30.73,20.19 | 36.83,14.61 36.81,14.62
  Top 0.305: 36.83,14.61 36.83,14.38 35.51,13.06 v35.51,12.04
  Bottom 0.254: 34.04,50.42 34.04,50.55 J2.12
  Bottom 0.381: 64.9,23.09 64.9,26.57
  Bottom 0.406: ICSP.4 66.18,27.83 64.9,26.57 | 64.9,23.09 65.79,22.23 65.79,17.02 63.25,14.48 48.39,14.48 42.85,8.94 38.56,8.94 37.21,10.29 v35.51,12.04 | 34.04,50.42 38.61,45.85 38.61,30.48 31.88,23.75 31.88,21.97 30.73,20.83 v30.73,20.19
MOSI2
  Top 0.254: TP_MOSI2.X 19.56,43.69 21.59,43.69 23.24,42.04 23.24,36.96 22.7,36.42 U3.16
N$1  (via drill 0.61)
  Top 0.279: RN2.1 26.61,40.57 25.53,41.66 TP_LL.X 26.67,42.16 L.A
  other vias: 25.53,43.18
N$3  (via drill 0.61)
  Top 0.305: RN4.6 56.62,34.18 56.39,34.42 56.39,35.31 | 56.39,35.31 56.39,35.94 ON.A | RN4.5 56.97,34.98 TP_ONL.X 56.39,35.31
  other vias: 56.64,35.05
N$4
  Top 0.254: U4.18 41.3,12.64
  Top 0.406: 41.3,12.64 41.1,12.45 | 40.23,10.87 39.95,10.87 C10.1
  Top 0.61: 41.1,12.45 41.1,11.73 40.23,10.87 | C10.1 39.7,7.93 L2.2
N$35  (via drill 0.61)
  Top 0.305: RX.A 28.96,34.29 28.96,34.42 30.23,35.69 TP_RXL.X 32.97,37.29 32.97,38.96 32.16,39.77 RN2.7
  other vias: 31.37,35.69
N$36  (via drill 0.61)
  Top 0.305: TX.A 29.25,36.57 30.8,36.57 31.75,37.52 31.75,38.35 v31.52,38.73 31.13,38.97 RN2.6
  Bottom 0.406: TP_TXL.X v31.52,38.73
PB4
  Top 0.279: U3.18 21.19,39.52
  Top 0.305: 21.19,39.52 JP2.1
PB5
  Top 0.279: 20.83,41.78 19.56,40.51 19.56,39.32 20.69,38.19 U3.19
  Top 0.305: 20.83,41.78 JP2.3
PB6
  Top 0.279: U3.20 20.19,37.88 18.29,39.73 JP2.2
PB7
  Top 0.279: 17.78,38.48 18.8,38.48 19.69,37.61 U3.21
  Top 0.305: JP2.4 18.29,41.78 17.02,40.51 17.02,39.24 17.78,38.48
PWRIN
  Top 0.813: D1.A 18.88,3.3 18.03,3.3 13.72,7.62 12.37,7.62 X1.2
  Bottom 0.813: X1.2 11.73,8.26
RD+
  Top 0.279: U3.29 16,34.42 14.35,36.07
  Top 0.305: 14.35,36.07 14.35,37.97 14.29,38.03 RN3.4
RD-
  Top 0.254: RN3.1 13.53,35.63
  Top 0.279: U3.30 15.34,33.92 RN3.1
RESET  (via drill 0.61)
  Top 0.254: U4.29 54.86,16.12 v59.56,20.83 60.2,20.83 63.63,24.26 ICSP.5
  Top 0.305: C5.2 28.83,29.46 27.18,27.81 RESET-EN.1
  Top 0.406: RESET-EN.2 RESET-EN.1 | J1.3 32.51,3.05 32.51,7.49 28.57,11.43 28.57,20.95 29.82,22.07 30.33,22.07 31.11,22.86 31.11,24.89 RESET-EN.2 | RN1.4 28.61,27.85 RESET-EN.2 | RESET.3 2.88,47.66 3.68,46.86 8,46.86 8.76,47.62 v8.89,47.66 RESET.4 | RESET-EN.2 30.23,28.83 v30.23,29.34 30.73,28.83 34.29,28.83 35.31,29.84 41.15,29.84 46.99,24 58.67,24 v59.44,24.77 D2.A
  Bottom 0.254: v8.89,47.66 9.89,48.67 10.05,48.64 12.7,48.64 15.11,46.23 16.38,46.23 17.02,46.86 17.02,48.01 17.8,48.79 21.87,48.79 23.93,46.74
  Bottom 0.305: 23.93,46.74 24.61,46.1 28.7,46.1 33.4,41.4 33.4,34.67 31.11,32.38 31.11,30.99 30.23,30.1 v30.23,29.34
  Bottom 0.406: v59.56,20.83 59.44,20.95 v59.44,24.77
RESET2  (via drill 0.61)
  Top 0.279: 16.85,37.12 U3.24
  Top 0.305: v22.61,46.61 22.61,47.62 21.46,48.77 17.02,48.77 TP_RESET2.X 13.51,47.5 D3.A 13.08,46.48 13,46.4 12.62,46.4 11.56,45.34 11.56,43.81 12.06,43.31 15.37,43.31 16.26,42.42 16.26,37.72 16.85,37.12
  Top 0.406: RN1.6 26.18,24.28 26.16,24.26 v25.84,24.53 v25.83,24.54
  Bottom 0.406: v22.61,46.61 22.86,46.35 22.86,44.58 23.88,43.56 23.88,42.29 24.38,41.78 25.53,41.78 26.14,41.17 26.14,40.18 24,38.05 24,30.23 26.16,28.07 26.16,24.87 v25.83,24.54
RXLED
  Top 0.279: RX.C 25.02,34.29 24.15,33.42 U3.10
SCK  (via drill 0.61)
  Top 0.254: U4.17 40.8,13.11 v39.78,12.14
  Top 0.305: v26.92,21.46 25.15,21.46 23.75,22.86 18.03,22.86 16.94,21.76 U5.5
  Bottom 0.254: 28.96,50.67 29.08,50.67 J2.14
  Bottom 0.406: ICSP.3 62.1,26.42 62.1,24.77 65.02,21.84 65.02,17.4 62.99,15.37 51.31,15.37 48.26,18.41 48.26,21.84 47.75,22.35 46.48,22.35 45.85,21.72 45.85,15.75 44.07,13.97 41.66,13.97 v39.78,12.14 38.73,12.14 37.72,13.21 37.72,14.22 36.58,15.37 30.73,15.37 27.81,18.29 27.81,20.07 26.92,20.95 v26.92,21.46 26.92,21.97 28.83,23.88 28.83,24.26 36.58,32 36.58,43.05 28.96,50.67
SCK2
  Top 0.254: U3.15 23.48,35.92 24,36.45 24,43.56 21.34,46.23 20.32,46.23 19.05,47.5 TP_SCK2.X
SS  (via drill 0.61)
  Top 0.254: U4.14 37.33,15.12 32.77,19.68 v32.77,20.95
  Bottom 0.254: 36.58,50.42 36.58,50.55 J2.11
  Bottom 0.406: 36.58,50.42 39.5,47.5 39.5,29.72 32.77,22.99 v32.77,20.95
TP_VUCAP  (via drill 0.61)
  Top 0.279: U3.27 16.98,35.42 15.62,36.78 | 15.62,40.51 15.62,41.27 TP_VUCAP.X C8.1
  Top 0.305: 15.62,36.78 15.62,40.51
  other vias: 14.99,41.91
TXLED
  Top 0.279: U3.11 23.51,33.92 26.16,36.58 TX.C
UGND
  Top 0.279: U3.28 16.51,34.92 14.99,36.45
  Top 0.305: 14.99,36.45 14.99,39.88 14.22,40.64
  Top 0.406: C8.2 11.81,41.27 12.45,40.64 14.22,40.64
  Top 0.61: L1.1 8.72,45 C8.2
  Top 0.813: L1.1 8.74,44.51 4.45,40.16 4.45,37.47 5.08,36.83 6.5,36.83 X2.4
  Bottom 0.61: X2.4 6.5,36.83
  Bottom 0.813: X2.4 5.06,36.85 4.45,37.47 4.45,40.01 5.71,41.27 10.03,41.27 GROUND.2
USBVCC  (via drill 0.61)
  Top 0.279: U3.31 16.78,33.42 16.64,33.27
  Top 0.406: 16.64,33.27 15.37,33.27 14.53,32.44 11.48,32.44 TP_USBVCC.X 9.91,28.96 10.54,28.32 10.54,27.18 9.88,26.52 T1.1
  Top 0.61: F1.1 3.47,24.51
  Top 0.813: 3.47,24.51 4.47,24.51 T1.1
  other vias: 9.91,30.86
USHIELD  (via drill 0.61)
  Top 0.61: TP_USH.X 9.02,42.67 11.7,39.99 Z1.2 | 11.06,33.54 11.19,33.54 11.3,33.66 Z2.2
  Top 0.813: L1.2 4.79,45.09 X2.P$1 | 11.06,33.54 5.25,33.54 X2.P$2
  Bottom 0.61: TP_USH.X 5.11,42.8 X2.P$1
  Bottom 0.813: X2.P$1 3.81,44.07 2.67,42.93 2.67,33.27 3.81,32.13 X2.P$2
  other vias: 9.02,42.8
VIN  (via drill 0.61)
  Top 0.305: RN1.8 24.82,22.68 24,23.5 17.53,23.5 15.24,21.21 15.24,19.3 14.8,18.86
  Top 0.61: 13.97,19.68 12.7,19.68 | 13.97,19.68 14.61,19.05 14.8,18.86 15.62,18.03 15.62,10.54 16.76,9.4 23.38,9.4 23.95,9.96 | 13.97,19.68 12.67,19.71 U1.3 | PC1.+ 25.54,11.43
  Top 0.813: v48.26,8.26 46.35,8.26 45.72,7.62 J1.8 | D1.C 23.79,9.81 23.95,9.96 PC1.+ 25.53,10.79 27.81,8.51 v27.81,8
  Bottom 0.813: v48.26,8.26 47.75,8.26 46.35,6.86 37.59,6.86 36.7,7.75 28.07,7.75 v27.81,8
XT1
  Top 0.254: R1.1 18.29,29.72
  Top 0.279: 18.19,29.75 U3.1
  Top 0.305: R1.1 18.19,29.75
  Top 0.406: C9.1 16.89,26.67 16.51,26.67 Y1.2
  Top 0.61: C9.1 R1.1
XT2
  Top 0.279: U3.2 18.69,30.84 R1.2
  Top 0.406: R1.2 C11.1 21.34,26.8 21.46,26.67 Y1.1
XTAL1
  Top 0.254: R2.1 42.16,20.57 42.55,20.19 41.66,20.19 41.3,19.83 U4.7
  Top 0.406: Y2.3 42.27,22.84 R2.1
XTAL2
  Top 0.254: R2.2 40.39,20.57 40.01,20.19 40.51,20.19 40.8,19.91 U4.8
  Top 0.406: Y2.1 40.27,22.84 R2.2
XUSB
  Top 0.813: F1.2 2.5,28.49 1.4,29.59 1.4,33.78 2.54,34.92 7.62,34.92 8.51,35.81 X2.1
  Bottom 0.305: X2.1 8.51,36.84

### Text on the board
Top: 3.325
Bottom: UNO SMD Rev3e
tPlace: 13 | 12 | 11 | 10 | 9 | 8 | 7 | 6 | 5 | 4 | 3 | 2 | 1 | 0 | MADE IN | ITALY
tNames: SCL | SDA | AREF | GND | # | # | # | # | # | # | DIGITAL | [#=PWM] | TX | RX | R | RN2 | Arduino | TX | RX | UNO | RN4 | Arduino | 1 | U5 | RN1 | ANALOG IN | IOREF | RESET | 3V3 | 5V | GND | VIN | A0 | A1 | A2 | A3 | A4 | A5
bNames: designed by | MADE IN | tinker it | ITALY
ReferenceLC: L | TX | ON | RX | PC1 | PC2
214bmp: D:/SmartProjects/Snc/a4_bn_logo2.bmp

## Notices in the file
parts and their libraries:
Arduino-utility: Copyright (c) 2016-2017 Arduino LLC. All right reserved.
Arduino-utility: This file is licensed under : CC-SA-BY-NC
